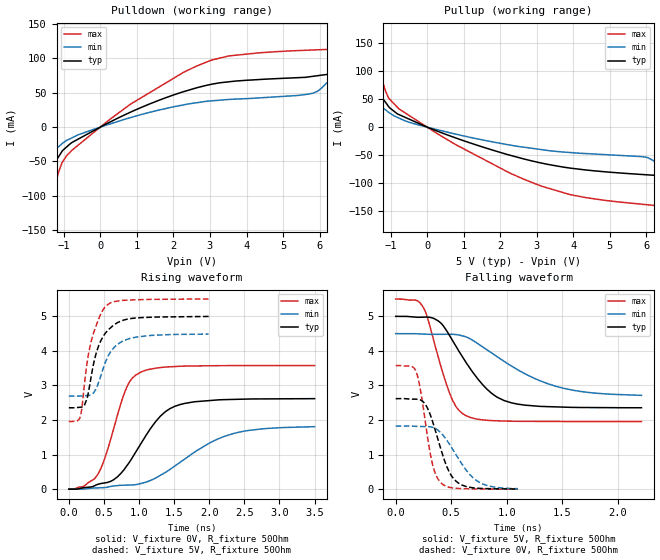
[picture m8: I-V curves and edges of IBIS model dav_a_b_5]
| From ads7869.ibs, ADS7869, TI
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|   dav_a_b_5 Model
[Model]   dav_a_b_5
Model_type   Output
Polarity   Non-Inverting
Vmeas = 2.5
Vref = 2.5
Cref = 30pF
Rref = 50
|   typ   min   max
|   (nom PVT)   (fast PVT)   (slow PVT)
|C_comp from frequency sweep method (F=8MHz)
|C_comp   3.418e-12   3.357e-12   3.518e-12
|ON state : BUFFER OUTPUT TURNED HIGH
|C_comp   3.418e-12   3.357e-12   3.518e-12
|OFF state: BUFFER OUTPUT TURNED LOW
|C_comp   3.082e-12   2.920e-12   3.216e-12
|C_comp from LC tank measurement(L=1nH)
|Resonant Frequency(Hz)   3.190e+09   3.210e+09   3.180e+09
C_comp   2.492e-12   2.461e-12   2.507e-12
|ON state : BUFFER OUTPUT TURNED HIGH
|Resonant Frequency(Hz)   3.190e+09   3.210e+09   3.180e+09
|C_comp   2.492e-12   2.461e-12   2.507e-12
|OFF state: BUFFER OUTPUT TURNED LOW
|Resonant Frequency(Hz)   3.280e+09   3.310e+09   3.230e+09
|C_comp   2.357e-12   2.314e-12   2.430e-12
| Where nom  PVT is Nominal Process, 5V, 36C
|   Fast PVT is Strong Process,  5.5V, -40C
|   Slow PVT is Weak Process,   4.5V, 96C
[Voltage Range]   5   4.5   5.5
|Ambient Temperature   25   85   -40
|Junction Temperature
[Temperature Range]   36   96   -40
[Pullup Reference]   5   4.5   5.5
[Pulldown Reference]   0   0   0
[Power Clamp Reference]   5   4.5   5.5
[GND Clamp Reference]   0   0   0
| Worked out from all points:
|   slope of the pulldown table from 0 to 0.75 V, typ, clamps not added: 37.5 ohm
|   slope of the pullup table from 0 to 0.75 V, typ, clamps not added: 40.1 ohm
|   falling waveform, V_fixture 5V, R_fixture 50Ohm: 20-80 % time 345ps typ, 583ps min, 199ps max; typ from 5 V to 2.36 V
|   rising waveform, V_fixture 0V, R_fixture 50Ohm: 20-80 % time 527ps typ, 846ps min, 327ps max; typ from 0 V to 2.62 V
|   rising waveform, V_fixture 5V, R_fixture 50Ohm: 20-80 % time 218ps typ, 241ps min, 197ps max; typ from 2.35 V to 5 V
|   falling waveform, V_fixture 0V, R_fixture 50Ohm: 20-80 % time 160ps typ, 232ps min, 109ps max; typ from 2.62 V to 0.007 V
[Pulldown]
|   Voltage   I(typ)   I(min)   I(max)
-5V       -424.9mA   -232mA     -913.5mA
-1.25V    -51.92mA   -33.42mA   -86.46mA
-924.5mV  -28.91mA   -19.36mA   -41.67mA
4mV       254.9uA    154.8uA    409.4uA
2.997V    61.95mA    38.12mA    96.72mA
5.697V    73.18mA    48.13mA    112.1mA
6.27V     77.41mA    68.35mA    113.4mA
6.465V    83.53mA    79.89mA    115.6mA
6.776V    112.4mA    98.26mA    118.9mA
6.941V    130.1mA    108mA      139.6mA
7.205V    158.4mA    123.6mA    198mA
10V       458mA      289.2mA    848.8mA
[Pullup]
|   Voltage   I(typ)   I(min)   I(max)
-5V       455.2mA    258.2mA    958.4mA
-1.25V    54.09mA    36.59mA    87.12mA
-1.056V   36.87mA    26.6mA     51.92mA
-608mV    17.63mA    11.34mA    25.69mA
758.5mV   -18.88mA   -12.2mA    -30.63mA
3.068V    -63.58mA   -39.76mA   -104.3mA
4.339V    -76.77mA   -47.34mA   -126.3mA
6.034V    -85.51mA   -54.57mA   -139.2mA
6.55V     -91.26mA   -78.05mA   -143.3mA
6.814V    -112.1mA   -91.99mA   -145.9mA
7.293V    -159.6mA   -117.2mA   -215.8mA
10V       -428.9mA   -260.3mA   -813.8mA
[Ramp]
R_load = 50
|   typ   min   max
dV/dt_r   1.57076/5.27093e-10   1.08471/8.4455e-10   2.14556/3.27456e-10
dV/dt_f   1.5874/3.45181e-10   1.08483/5.95988e-10   2.12526/1.98679e-10
[Falling Waveform]
V_fixture = 5V
V_fixture_min = 4.5V
V_fixture_max = 5.5V
R_fixture = 50Ohm
|   Time   V(typ)   V(min)   V(max)
0s        5V         4.5V       5.5V
181.1ps   4.977V     4.497V     5.468V
250.2ps   4.977V     4.488V     5.251V
380.9ps   4.873V     4.48V      3.852V
482.7ps   4.46V      4.482V     2.805V
624.8ps   3.712V     4.414V     2.142V
826.8ps   2.881V     4.022V     1.993V
1.045ns   2.496V     3.558V     1.967V
1.521ns   2.374V     2.913V     1.959V
2.214ns   2.356V     2.715V     1.958V
[Rising Waveform]
V_fixture = 0V
V_fixture_min = 0V
V_fixture_max = 0V
R_fixture = 50Ohm
|   Time   V(typ)   V(min)   V(max)
0s        1.045nV    10.66nV    945.3pV
219.2ps   44.34mV    7.391mV    90.13mV
406.2ps   134.1mV    37.49mV    407.6mV
512.1ps   181.1mV    45.27mV    892.1mV
822.8ps   665.9mV    117.2mV    2.94V
1.019ns   1.291V     160.2mV    3.379V
1.305ns   2.113V     401.3mV    3.518V
1.582ns   2.446V     772.6mV    3.555V
2.354ns   2.597V     1.615V     3.574V
3.5ns     2.618V     1.808V     3.576V
[Rising Waveform]
V_fixture = 5V
V_fixture_min = 4.5V
V_fixture_max = 5.5V
R_fixture = 50Ohm
|   Time   V(typ)   V(min)   V(max)
0s        2.354V     2.691V     1.958V
156.5ps   2.369V     2.694V     2.055V
181.1ps   2.374V     2.697V     2.276V
220.1ps   2.416V     2.703V     2.989V
305.2ps   3.099V     2.722V     4.161V
411.1ps   4.069V     3.015V     4.849V
539.9ps   4.559V     3.764V     5.318V
668.7ps   4.786V     4.146V     5.433V
872.3ps   4.931V     4.361V     5.473V
1.992ns   4.996V     4.485V     5.499V
[Falling Waveform]
V_fixture = 0V
V_fixture_min = 0V
V_fixture_max = 0V
R_fixture = 50Ohm
|   Time   V(typ)   V(min)   V(max)
0s        2.619V     1.825V     3.576V
181.1ps   2.605V     1.819V     3.425V
219.2ps   2.588V     1.814V     2.942V
322.2ps   2.058V     1.798V     853.5mV
365.3ps   1.611V     1.741V     393.3mV
406.2ps   1.169V     1.635V     188.1mV
502ps     390.8mV    1.214V     43mV
596.3ps   120.7mV    731.5mV    17.35mV
785.2ps   20.39mV    149.8mV    5.78mV
1.101ns   6.845mV    15.45mV    1.396mV
